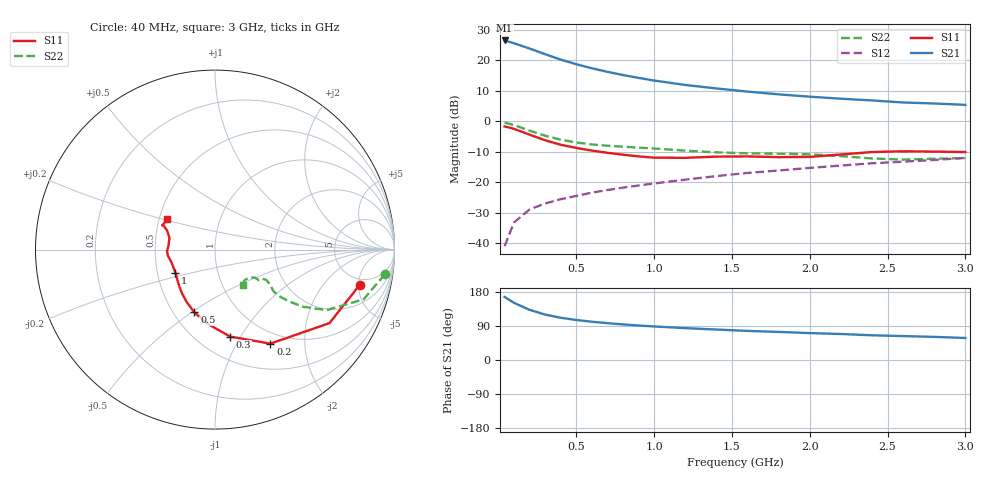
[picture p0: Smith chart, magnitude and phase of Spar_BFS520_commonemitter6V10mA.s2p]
! Filename:  BFS520I.S2P  Version:  4.0
! NXP part #: BFS520  Date: Jun 1994
! Bias condition: Vce=6V, Ic=10mA
#  MHz  S  MA  R  50
! Freq  S11  S21  S12  S22  !GUM [dB]
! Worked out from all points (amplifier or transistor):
!   21 points, 40 MHz to 3 GHz, reference 50 ohm
!   highest |S21| = 26.6 dB at 40 MHz (marker M1)
!   |S21| within 3 dB of that: start of sweep to 219.1 MHz
!   unconditionally stable (mu >= 1): 875.7 MHz to end of sweep
!   at 300 MHz: K = 0.61, MSG = 24.5 dB, |S12| = -26.9 dB
!   at 1 GHz: K = 1.04, MAG = 15.6 dB, |S12| = -20.4 dB
!   at 3 GHz: K = 1.06, MAG = 7.2 dB, |S12| = -12.0 dB
!   lowest NFmin = 1.10 dB at 500 MHz
!   S11 on the Smith chart (normalised r, x): 40 MHz: 4.09, -5.16; 200 MHz: 0.84, -1.39; 300 MHz: 0.71, -0.90; 500 MHz: 0.63, -0.51; 1 GHz: 0.62, -0.17; 3 GHz: 0.55, +0.21
40  0.83 -13.7  21.31 166.3  0.009 82.2  0.957 -8.2
100  0.758 -32.7  19.2 151.0  0.022 72.8  0.873 -18.5
200  0.608 -59.5  15.71 132.4  0.036 63.4  0.707 -28.5
300  0.492 -80.1  12.68 119.9  0.045 60.5  0.584 -33.0
400  0.415 -95.9  10.35 111.5  0.053 60.1  0.503 -35.0
500  0.368 -108.2  8.684 105.6  0.06 60.9  0.452 -35.8
600  0.333 -118.1  7.455 101.0  0.068 62.3  0.42 -35.8
700  0.306 -126.8  6.519 97.2  0.075 63.8  0.4 -35.4
800  0.285 -134.4  5.778 93.9  0.082 64.9  0.386 -34.4
900  0.267 -142.1  5.184 91.0  0.089 66.0  0.372 -33.3
1000  0.255 -149.9  4.689 88.5  0.096 66.8  0.36 -32.2
1200  0.253 -164.0  3.971 84.1  0.111 68.2  0.332 -30.6
1400  0.265 -172.8  3.479 80.4  0.127 69.4  0.311 -31.5
1600  0.267 -178.4  3.09 76.8  0.143 69.5  0.3 -34.3
1800  0.26 175.5  2.782 74.1  0.157 70.3  0.296 -35.1
2000  0.262 165.7  2.547 71.0  0.173 70.4  0.289 -34.7
2200  0.287 158.3  2.362 68.6  0.189 70.8  0.27 -35.2
2400  0.315 155.1  2.211 65.2  0.206 70.6  0.247 -39.0
2600  0.324 155.3  2.047 63.1  0.219 70.0  0.237 -45.8
2800  0.32 153.4  1.97 61.0  0.234 70.3  0.245 -50.5
3000  0.315 147.5  1.871 58.1  0.252 69.9  0.251 -52.0
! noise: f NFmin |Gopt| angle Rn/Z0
500  1.1  0.25  48  0.23
900  1.25  0.21  49  0.23
2000  1.9  0.23  162  0.15
